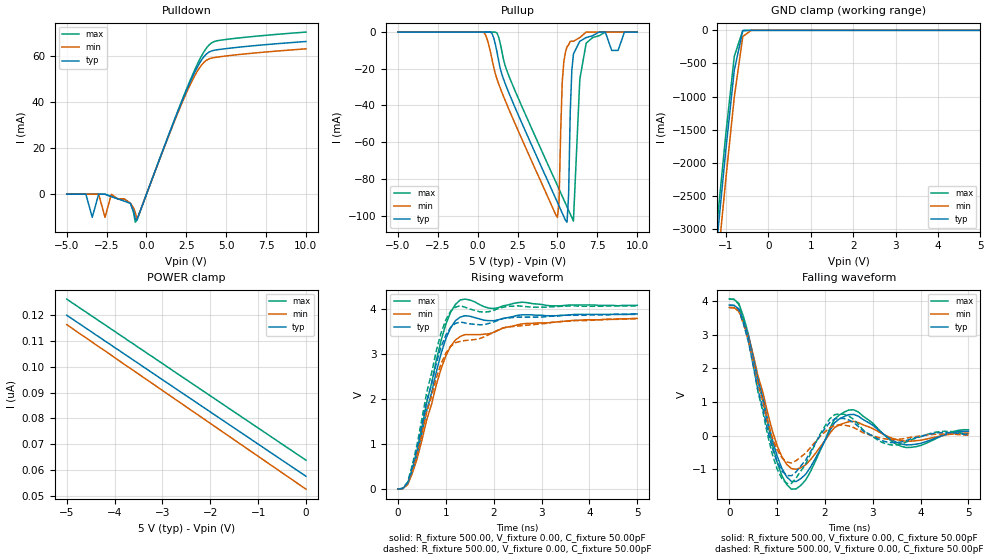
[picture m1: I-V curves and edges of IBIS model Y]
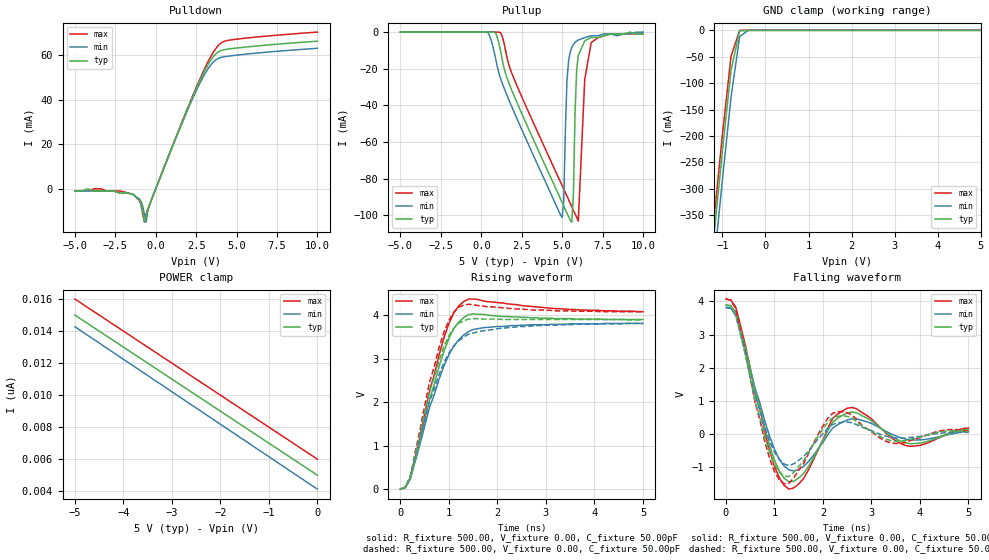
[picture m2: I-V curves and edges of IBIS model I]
| IBIS file qs3251.ibs
[IBIS ver]   2.1
[File name]   qs3251.ibs
[File Rev]   1.0
[Date]   January 24, 1996
[Source]   From QSI silicon model
[Notes]   QSI provides IBIS models as a service to our customers. You
   and your company shall not distribute, convey, sell or give
   these models to anyone else without receiving prior written
   permission from QSI. QSI reserves the right to make changes to
   its products or to discontinue any semiconductor product or
   service without notice, and advises its customers to obtain
   the latest version of relevant information to verify, before
   placing orders, that the information being relied on is
   current. Please be aware that your receipt and subsequent use
   of the IBIS information provided shall serve as acceptance of
   the terms and conditions of this agreement. If you do not
   accept these terms, you should return the IBIS model and any
   other accompanying information immediately.
[Disclaimer] PLEASE BE AWARE THAT IN THE ABSENCE OF A SIGNED, WRITTEN
   AGREEMENT TO THE CONTRARY, Quality Semiconductor Incorporated
   ("QSI") IS PROVIDING THIS IBIS MODEL AS IS" AND WITHOUT AND
   WARRANTY, EXPRESSED OR IMPLIED. Further, QSI assumes no
   liability for: 1) the accuracy of the IBIS models provided to
   your company; 2) the proper functioning of these IBIS models
   in your design or for any resulting applications; or 3)
   infringement of patents, copyrights or intellectual property
   rights resulting from your use of these IBIS models. These
   commodities, technical data, and software may be U.S. export
   license controlled. As such, prior to export or re-export,
   U.S. Government approval and authorization may be required.
[Copyright]   (C) Copyright 1996 Quality Semiconductor Incorporated. All
   rights reserved. Unauthorized reproduction and/or distribution
   is strictly prohibited.
|   Component qs3251
[Component]   qs3251
[Manufacturer]   Quality Semiconductor Incorporated
[Package]
| Note that R_pkg is not given
| variable   typ   min   max
| Package parasitics.  Uncomment one set.
| SOIC (150)
R_pkg   0.00   0.00   0.00
L_pkg   3.00nH   NA   NA
C_pkg   600.00fF   NA   NA
| QSOP
|R_pkg   0.00   0.00   0.00
|L_pkg   2.50nH   NA   NA
|C_pkg   0.40pF   NA   NA
[Pin]  signal_name   model_name   R_pin   L_pin   C_pin
1   I3   I
2   I2   I
3   I1   I
4   I0   I
5   Y   Y
6   NC   NC
|7   E   EnableA
8   GND   GND
|9   S2   SelectA
|10   S1   SelectA
|11   S0   SelectA
12   I7   I
13   I6   I
14   I5   I
15   I4   I
16   Vcc   POWER
| Models and submodels in the file (2): Y (3-state), I (3-state)
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|   Model Y
[Model]   Y
Model_type   3-state
Vinl =   0.00V
Vinh =   5.00V
C_comp   5.00pF   5.00pF   5.00pF
[Temperature Range]   25.00   70.00   0.00
[Voltage Range]   5.00V   4.50V   5.50V
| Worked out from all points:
|   slope of the pulldown table from 0 to 0.75 V, typ, clamps not added: 54 ohm
|   GND clamp passes 1 mA (typ) near -0.43 V on its own axis
|   rising waveform, R_fixture 500.00, V_fixture 0.00, C_fixture 50.00pF: 20-80 % time 532ps typ, 615ps min, 505ps max; typ from 0 V to 3.89 V
|   rising waveform, R_fixture 500.00, V_fixture 0.00, C_fixture 50.00pF: 20-80 % time 515ps typ, 609ps min, 487ps max; typ from 0 V to 3.88 V
|   falling waveform, R_fixture 500.00, V_fixture 0.00, C_fixture 50.00pF: 20-80 % time 380ps typ, 401ps min, 370ps max; typ from 3.89 V to 0.128 V
|   falling waveform, R_fixture 500.00, V_fixture 0.00, C_fixture 50.00pF: 20-80 % time 365ps typ, 390ps min, 352ps max; typ from 3.89 V to 0.023 V
[Pulldown]
| voltage   I(typ)   I(min)   I(max)
-5V       0A         0A         0A
-3.8V     0A         0A         0A
-3.4V     -10mA      0A         0A
-3V       0A         0A         0A
-2.6V     0A         -10mA      0A
-2.2V     -1mA       0A         -1mA
-1.4V     -3mA       -2mA       -2mA
-700mV    -10.8mA    -8.1mA     -12.14mA
-500mV    -9.35mA    -9.33mA    -9.38mA
2.7V      48.06mA    46.93mA    48.77mA
3.9V      61.6mA     58.65mA    64.59mA
10V       66.28mA    63.1mA     70.37mA
[Pullup]
| voltage   I(typ)   I(min)   I(max)
-5V       0A         0A         0A
400mV     0A         -287.4uA   0A
1.2V      -10.52mA   -25.42mA   -411.1uA
5V        -92.88mA   -101mA     -83.69mA
5.1V      -94.82mA   -92.21mA   -85.62mA
5.3V      -98.68mA   -27mA      -89.48mA
5.6V      -103.6mA   -8mA       -95.26mA
5.8V      -43.8mA    -5mA       -99.11mA
6V        -12mA      -5mA       -103mA
6.4V      -5mA       -3mA       -25.8mA
6.8V      -3mA       0A         -6mA
10V       0A         0A         0A
[GND_clamp]
| voltage   I(typ)   I(min)   I(max)
-5V       -29.56A    -29.97A    -29.34A
-1.4V     -4.48A     -4.92A     -4.23A
-1.2V     -3.13A     -3.57A     -2.88A
-1V       -1.81A     -2.25A     -1.57A
-800mV    -602.4mA   -1.01A     -393mA
-600mV    -6.68mA    -93.98mA   -834.9uA
-400mV    -2.89uA    -170.1uA   -176.2nA
5V        62.5nA     63.88nA    62.5nA
[POWER_clamp]
| voltage   I(typ)   I(min)   I(max)
-5V       120nA      116.4nA    126.3nA
-4.7V     116.3nA    112.5nA    122.5nA
-4.2V     110nA      106.2nA    116.3nA
0V        57.5nA     52.49nA    63.75nA
[Ramp]
| variable   typ   min   max
dV/dt_r   2.34/236.24p   2.29/284.78p   2.44/205.22p
dV/dt_f   2.98/100.00p   2.68/150.00p   3.28/100.00p
[Rising Waveform]
R_fixture = 500.00
V_fixture = 0.00
C_fixture = 50.00pF
L_dut = 3.00nH
C_dut = 600.00fF
| time   V(typ)   V(min)   V(max)
0s        0V         0V         0V
200ps     116.9mV    97.73mV    131.4mV
400ps     783.6mV    677.5mV    869.9mV
600ps     1.75V      1.54V      1.93V
900ps     3.01V      2.67V      3.3V
1.1ns     3.58V      3.17V      3.93V
1.3ns     3.82V      3.39V      4.2V
2ns       3.74V      3.48V      4.01V
2.6ns     3.87V      3.67V      4.15V
5ns       3.89V      3.79V      4.08V
[Rising Waveform]
R_fixture = 500.00
V_fixture = 0.00
C_fixture = 50.00pF
L_dut = 2.50nH
C_dut = 400.00fF
| time   V(typ)   V(min)   V(max)
0s        0V         0V         0V
200ps     138.5mV    115.8mV    155.8mV
400ps     904.4mV    781.2mV    1V
600ps     1.95V      1.71V      2.15V
900ps     3.16V      2.79V      3.47V
1ns       3.42V      3.02V      3.76V
1.2ns     3.68V      3.25V      4.04V
1.8ns     3.65V      3.38V      3.93V
2.3ns     3.8V       3.6V       4.06V
5ns       3.88V      3.78V      4.07V
[Falling Waveform]
R_fixture = 500.00
V_fixture = 0.00
C_fixture = 50.00pF
L_dut = 3.00nH
C_dut = 600.00fF
| time   V(typ)   V(min)   V(max)
0s        3.89V      3.82V      4.07V
200ps     3.78V      3.72V      3.94V
300ps     3.41V      3.4V       3.53V
1ns       -611.1mV   -299.8mV   -797mV
1.3ns     -1.37V     -986mV     -1.6V
1.6ns     -1.15V     -870mV     -1.32V
2.2ns     382.9mV    236.9mV    484.9mV
2.5ns     622.4mV    412.1mV    761.7mV
3.7ns     -279.8mV   -169.5mV   -358.2mV
5ns       128.4mV    70mV       172.2mV
[Falling Waveform]
R_fixture = 500.00
V_fixture = 0.00
C_fixture = 50.00pF
L_dut = 2.50nH
C_dut = 400.00fF
| time   V(typ)   V(min)   V(max)
0s        3.89V      3.82V      4.07V
200ps     3.76V      3.7V       3.91V
400ps     2.79V      2.83V      2.84V
900ps     -377mV     -61mV      -558.2mV
1.2ns     -1.19V     -789.3mV   -1.43V
1.4ns     -1.08V     -747.3mV   -1.26V
2.2ns     491.8mV    297.8mV    620.2mV
3.4ns     -213.1mV   -117.7mV   -281.4mV
4.4ns     84.76mV    43.07mV    116.9mV
5ns       23.44mV    9.28mV     34.24mV
|   Model I
[Model]   I
Model_type   3-state
Vinl =   0.00V
Vinh =   5.00V
C_comp   5.00pF   5.00pF   5.00pF
[Temperature Range]   25.00   70.00   0.00
[Voltage Range]   5.00V   4.50V   5.50V
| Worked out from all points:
|   slope of the pulldown table from 0 to 0.75 V, typ, clamps not added: 54 ohm
|   GND clamp passes 1 mA (typ) near -0.60 V on its own axis
|   rising waveform, R_fixture 500.00, V_fixture 0.00, C_fixture 50.00pF: 20-80 % time 559ps typ, 647ps min, 522ps max; typ from 0 V to 3.9 V
|   rising waveform, R_fixture 500.00, V_fixture 0.00, C_fixture 50.00pF: 20-80 % time 543ps typ, 647ps min, 500ps max; typ from 0 V to 3.89 V
|   falling waveform, R_fixture 500.00, V_fixture 0.00, C_fixture 50.00pF: 20-80 % time 379ps typ, 415ps min, 362ps max; typ from 3.89 V to 0.131 V
|   falling waveform, R_fixture 500.00, V_fixture 0.00, C_fixture 50.00pF: 20-80 % time 351ps typ, 393ps min, 334ps max; typ from 3.89 V to 0.066 V
[Pulldown]
| voltage   I(typ)   I(min)   I(max)
-5V       -1mA       -1mA       -1mA
-3.4V     -1mA       -1mA       0A
-1.4V     -2.6mA     -2.6mA     -2.5mA
-1V       -5.1mA     -4.6mA     -5.4mA
-800mV    -10.06mA   -7.9mA     -11.63mA
-700mV    -14.92mA   -11.6mA    -14.98mA
-600mV    -12.17mA   -15mA      -11.39mA
-300mV    -5.6mA     -5.56mA    -5.62mA
2.6V      46.47mA    45.45mA    47.11mA
3.3V      56.53mA    54.59mA    57.98mA
3.9V      61.6mA     58.65mA    64.59mA
10V       66.28mA    63.1mA     70.37mA
[Pullup]
| voltage   I(typ)   I(min)   I(max)
-5V       0A         0A         0A
400mV     0A         -287.5uA   0A
1.2V      -10.52mA   -25.42mA   -411.2uA
5V        -92.88mA   -101.1mA   -83.69mA
5.1V      -94.82mA   -92.15mA   -85.62mA
5.3V      -98.68mA   -26.3mA    -89.48mA
5.6V      -103.7mA   -8.4mA     -95.26mA
5.9V      -20.7mA    -4.9mA     -101mA
6V        -12.7mA    -4.3mA     -103mA
6.4V      -4.8mA     -3mA       -25.7mA
6.8V      -2.9mA     -2mA       -5.7mA
10V       -1mA       0A         -1mA
[GND_clamp]
| voltage   I(typ)   I(min)   I(max)
-5V       -3.69A     -3.75A     -3.67A
-1.4V     -559.6mA   -614.8mA   -529.2mA
-1.2V     -391.1mA   -446.6mA   -360.6mA
-1V       -226.9mA   -282mA     -196.7mA
-800mV    -75.3mA    -126.3mA   -49.05mA
-600mV    -834.8uA   -11.75mA   -104.4uA
-400mV    -361.2nA   -21.26uA   -22.2nA
5V        10nA       10.14nA    10nA
[POWER_clamp]
| voltage   I(typ)   I(min)   I(max)
-5V       15nA       14.27nA    16nA
-1V       7nA        6.16nA     8nA
-600mV    6.2nA      5.34nA     7.2nA
0V        5nA        4.13nA     6nA
[Ramp]
| variable   typ   min   max
dV/dt_r   2.34/78.60p   2.29/81.25p   2.44/73.59p
dV/dt_f   2.98/50.00p   2.68/50.00p   3.28/50.00p
[Rising Waveform]
R_fixture = 500.00
V_fixture = 0.00
C_fixture = 50.00pF
L_dut = 3.00nH
C_dut = 600.00fF
| time   V(typ)   V(min)   V(max)
0s        0V         0V         0V
100ps     39.97mV    36.63mV    36.51mV
200ps     240.7mV    218.7mV    242.2mV
600ps     2.07V      1.88V      2.26V
900ps     3.18V      2.84V      3.49V
1.1ns     3.69V      3.29V      4.05V
1.3ns     3.94V      3.54V      4.31V
1.5ns     4.03V      3.67V      4.37V
2ns       3.98V      3.74V      4.29V
5ns       3.9V       3.81V      4.08V
[Rising Waveform]
R_fixture = 500.00
V_fixture = 0.00
C_fixture = 50.00pF
L_dut = 2.50nH
C_dut = 400.00fF
| time   V(typ)   V(min)   V(max)
0s        0V         0V         0V
100ps     47.32mV    43.3mV     43.51mV
200ps     280.7mV    254.5mV    284mV
600ps     2.25V      2.02V      2.46V
900ps     3.29V      2.92V      3.62V
1.1ns     3.7V       3.29V      4.07V
1.2ns     3.81V      3.41V      4.18V
1.4ns     3.91V      3.56V      4.25V
2ns       3.91V      3.69V      4.18V
5ns       3.89V      3.81V      4.08V
[Falling Waveform]
R_fixture = 500.00
V_fixture = 0.00
C_fixture = 50.00pF
L_dut = 3.00nH
C_dut = 600.00fF
| time   V(typ)   V(min)   V(max)
0s        3.89V      3.82V      4.07V
200ps     3.66V      3.6V       3.83V
900ps     -356.5mV   -79.63mV   -506.6mV
1.1ns     -1.12V     -767mV     -1.33V
1.3ns     -1.45V     -1.09V     -1.67V
1.6ns     -1.2V      -984mV     -1.35V
2.2ns     350.6mV    176.3mV    461.4mV
2.5ns     632.6mV    419.1mV    773mV
3.7ns     -272.5mV   -158.5mV   -352.1mV
5ns       130.8mV    70.09mV    176.1mV
[Falling Waveform]
R_fixture = 500.00
V_fixture = 0.00
C_fixture = 50.00pF
L_dut = 2.50nH
C_dut = 400.00fF
| time   V(typ)   V(min)   V(max)
0s        3.89V      3.82V      4.07V
200ps     3.62V      3.57V      3.78V
800ps     -81.32mV   200.1mV    -224.8mV
1ns       -924mV     -549.4mV   -1.14V
1.2ns     -1.28V     -912mV     -1.51V
1.6ns     -812mV     -685.8mV   -898.1mV
2.1ns     353.5mV    170mV      470.3mV
2.3ns     531.2mV    328.5mV    665.8mV
3.4ns     -202mV     -103.3mV   -272mV
5ns       65.57mV    40.78mV    83.15mV
